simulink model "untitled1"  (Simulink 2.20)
settings: Solver=ode45  StartTime=0.0  StopTime=10.0  RelTol=1e-3  AbsTol=1e-6

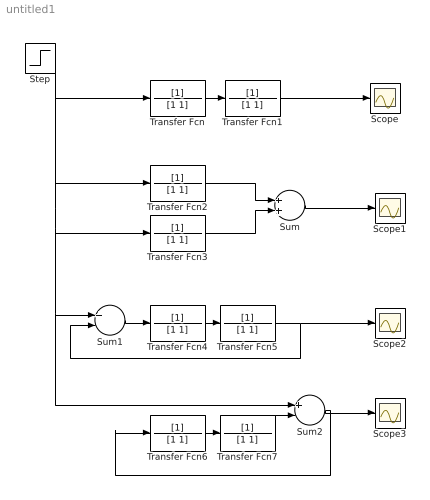
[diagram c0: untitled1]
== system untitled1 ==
  Scope{,1..3} (4 alike) : Scope
  Step : Step  Time=0  Before=0  After=1
  Sum : Sum  Inputs=++
  Sum1 : Sum  Inputs=+-
  Sum2 : Sum  Inputs=+-
  Transfer Fcn{,1..7} (8 alike) : TransferFcn  Numerator=[1]  Denominator=[1 1]
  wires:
  Step/1 -> Transfer Fcn2/1, Transfer Fcn/1, Transfer Fcn3/1, Sum1/1, Sum2/1
  Sum1/1 -> Transfer Fcn4/1
  Transfer Fcn4/1 -> Transfer Fcn5/1
  Transfer Fcn5/1 -> Sum1/2, Scope2/1
  Sum/1 -> Scope1/1
  Transfer Fcn7/1 -> Sum2/2
  Sum2/1 -> Transfer Fcn6/1, Scope3/1
  Transfer Fcn2/1 -> Sum/1
  Transfer Fcn3/1 -> Sum/2
  Transfer Fcn/1 -> Transfer Fcn1/1
  Transfer Fcn1/1 -> Scope/1
  Transfer Fcn6/1 -> Transfer Fcn7/1
